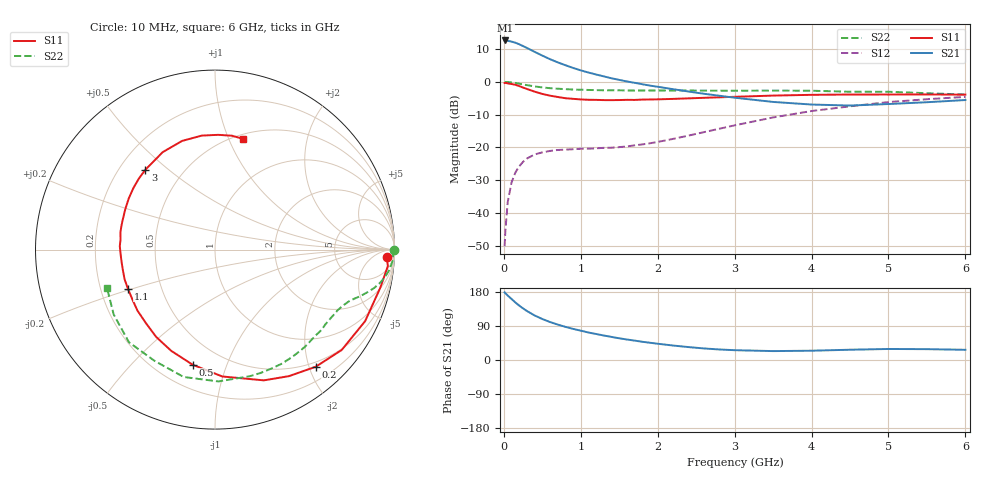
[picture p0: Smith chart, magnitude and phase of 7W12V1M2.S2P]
! Infineon Technologies  Discrete & RF Semiconductors
! BFS17W
! Si NPN RF Bipolar Junction Transistor in SOT323
! VCE = 12 V  IC = 1.2 mA
! Common Emitter S-Parameters:  August  1999
# GHz  S  MA  R  50
!  f  S11  S21  S12  S22
! GHz  MAG  ANG  MAG  ANG  MAG  ANG  MAG  ANG
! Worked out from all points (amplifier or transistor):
!   36 points, 10 MHz to 6 GHz, reference 50 ohm
!   highest |S21| = 12.6 dB at 20 MHz (marker M1)
!   |S21| within 3 dB of that: start of sweep to 360.3 MHz
!   unconditionally stable (mu >= 1): 1.032 GHz to 2.84 GHz; 4.266 GHz to end of sweep
!   at 250 MHz: K = 0.27, MSG = 17.7 dB, |S12| = -24.4 dB
!   at 1.4 GHz: K = 1.24, MAG = 7.7 dB, |S12| = -20.1 dB
!   at 6 GHz: K = 1.07, MAG = -2.1 dB, |S12| = -4.6 dB
!   S11 on the Smith chart (normalised r, x): 10 MHz: 23, -23; 200 MHz: 0.42, -2.11; 500 MHz: 0.34, -0.77; 1.1 GHz: 0.32, -0.19; 3 GHz: 0.31, +0.42; 6 GHz: 0.55, +1.13
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0.01  0.9573 -2.5  4.254 178.6  0.0031 89.1  0.9999 -0.2
0.02  0.9677 -5.4  4.277 176.2  0.0053 89.7  0.9926 -1.3
0.05  0.9451 -13.0  4.225 170.2  0.0145 83.1  0.9931 -3.3
0.1  0.9266 -25.5  4.108 161.1  0.0291 75.1  0.9795 -6.4
0.15  0.9005 -38.4  3.948 151.8  0.0412 68.9  0.9594 -9.2
0.2  0.8608 -49.3  3.744 143.6  0.0514 63.9  0.9367 -11.5
0.25  0.8166 -59.7  3.507 136.1  0.0601 57.8  0.9129 -13.5
0.3  0.7777 -69.5  3.291 129.3  0.0675 54.4  0.8903 -15.1
0.4  0.7081 -86.7  2.866 117.5  0.0778 47.4  0.8509 -17.7
0.5  0.6533 -101.0  2.512 108.2  0.0838 43.4  0.8214 -19.5
0.6  0.6145 -113.4  2.215 100.2  0.0881 40.5  0.7991 -21.2
0.7  0.5866 -124.0  1.982 93.5  0.0911 39.5  0.7843 -22.9
0.9  0.5497 -141.8  1.629 82.1  0.0935 38.6  0.7621 -26.3
1.1  0.5317 -155.9  1.386 72.5  0.0954 40.6  0.7511 -29.9
1.6  0.5308 177.9  1.012 54.1  0.1032 50.6  0.7373 -40.2
2.2  0.5485 155.6  0.771 38.2  0.1345 65.9  0.7368 -54.3
3  0.5902 131.2  0.572 25.9  0.2165 73.2  0.7315 -74.6
3.5  0.6163 118.2  0.493 23.5  0.2859 71.5  0.7348 -88.5
4  0.6327 106.8  0.45 24.5  0.358 66.2  0.7309 -103.8
4.5  0.6394 96.6  0.434 27.1  0.4225 59.6  0.7053 -118.7
5.5  0.6415 81.5  0.488 28.6  0.5426 45.3  0.6703 -147.4
6  0.6366 75.7  0.527 26.9  0.5888 38.4  0.6387 -160.3
